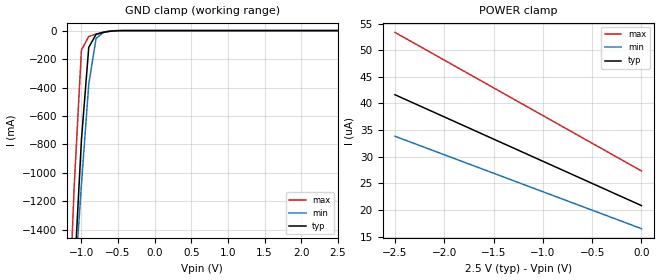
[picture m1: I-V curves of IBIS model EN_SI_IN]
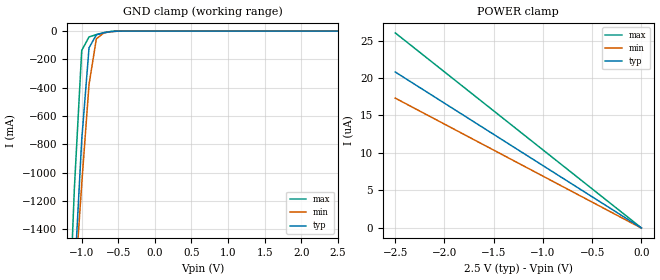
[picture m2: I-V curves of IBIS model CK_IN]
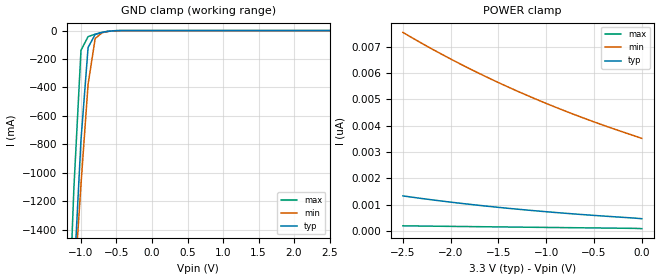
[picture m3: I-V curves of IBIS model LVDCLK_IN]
|   Texas Instruments Incorporated
|   IBIS Model for CDCLVD110A
|   32-PIN LQFP Package
[IBIS Ver]   3.2
[Comment char]   |_char
[File name]   cdclvd110a.ibs
[File Rev]   1.3   | pre-silicon, correlated to first silicon samples
[Date]   17Apr02
[Source]   File originated at Texas Instruments Incorporated.
   HPA HIGH SPEED COMMUNICATION AND CONTROLL, HSCC.
[Notes]   REVISION HISTORY:
   1.0: 03/26/02 initially release  version.
   1.1: 04/05/02 improved accuracy of rising/falling waveforms to solve
   warning messages during file check.
   Synchronized wave form data to match time with TPD
   (0ns = cross point at input)
   1.2: 04/17/02 Reviewed range completeness of I-V tables.
   1.3: 08/19/02 Corrected Warning on C_comp.
[Disclaimer]
(C) Copyright Texas Instruments Incorporated 2002
   All rights reserved
  Texas Instruments Incorporated hereby grants the user of this IBIS
model a non-exclusive, nontransferable license to use this IBIS model
under the following terms.  Before using this IBIS model, the user
should read this license.  If the user does not accept these terms,
the IBIS model should be returned to Texas Instruments within 30 days.
  The user is granted this license only to use the IBIS model and
is not granted rights to sell, load, rent, lease or license the IBIS
model in whole or in part, or in modified form to anyone other than
user.  User may modify the IBIS model to suit its specific applications
but rights to derivative works and such modifications shall belong to
Texas Instruments.
  This IBIS model is provided on an "AS IS" basis and Texas Instruments
makes absolutely no warranty with respect to the information contained
herein.  TEXAS INSTRUMENTS DISCLAIMS AND CUSTOMER WAIVES ALL WARRANTIES,
EXPRESS OR IMPLIED, INCLUDING WARRANTIES OF MERCHANTABILITY OR FITNESS
FOR A PARTICULAR PURPOSE. The entire risk as to quality and performance
is with the Customer. ACCORDINGLY, IN NO EVENT SHALL THE COMPANY BE LIABLE
FOR ANY DAMAGES, WHETHER IN CONTRACT OR TORT,INCLUDING ANY LOST PROFITS
OR OTHER INCIDENTAL, CONSEQUENTIAL, EXEMPLARY, OR PUNITIVE DAMAGES ARISING
OUT OF THE USE OR APPLICATION OF THE IBIS model provided in this package.
Further, Texas Instruments reserves the right to discontinue or make changes
without notice to any product herein to improve reliability, function, or
design. Texas Instruments does not convey any license under patent rights
or any other intellectual property rights, including those of third parties.
Contact Texas Instruments at ATTN: HPA-High Speed Communication & Control, HSCC
[Copyright]   Copyright 2002, Texas Instruments, All Rights Reserved
[Component]   CDCLVD110AVF
[Manufacturer]  Texas Instruments Incorporated
[Package]
|   typ   min   max
R_pkg   0.1026   0.0423   0.1248
L_pkg   3.424nH   2.117nH   4.030nH
C_pkg   0.276pF   0.217pF   0.610pF
[Pin] signal_name   model_name   R_pin   L_pin   C_pin
1   CK   CK_IN   0.1223   3.968nH   0.353pF
2   SI   EN_SI_IN   0.1106   3.670nH   0.268pF
3   CLK0_T   LVDCLK_IN   0.1043   3.429nH   0.235pF
4   CLK0_N   LVDCLK_IN   0.1018   3.304nH   0.218pF
5   VREF   NC   0.1022   3.313nH   0.218pF
6   CLK1_T   LVDCLK_IN   0.1054   3.453nH   0.228pF
7   CLK1_N   LVDCLK_IN   0.1129   3.696nH   0.247pF
8   EN   EN_SI_IN   0.1248   4.030nH   0.218pF
9   VSS   GND   0.0621   2.573nH   0.514pF
10   Q9_N   LVDCLK_OUT   0.1132   3.725nH   0.261pF
11   Q9_T   LVDCLK_OUT   0.1072   3.492nH   0.235pF
12   Q8_N   LVDCLK_OUT   0.1048   3.371nH   0.219pF
13   Q8_T   LVDCLK_OUT   0.1053   3.380nH   0.221pF
14   Q7_N   LVDCLK_OUT   0.1083   3.516nH   0.230pF
15   Q7_T   LVDCLK_OUT   0.1148   3.750nH   0.253pF
16   VDD   POWER   0.0424   2.117nH   0.476pF
17   Q6_N   LVDCLK_OUT   0.1235   3.997nH   0.288pF
18   Q6_T   LVDCLK_OUT   0.1116   3.673nH   0.265pF
19   Q5_N   LVDCLK_OUT   0.1048   3.439nH   0.234pF
20   Q5_T   LVDCLK_OUT   0.1020   3.309nH   0.219pF
21   Q4_N   LVDCLK_OUT   0.1020   3.308nH   0.217pF
22   Q4_T   LVDCLK_OUT   0.1047   3.440nH   0.227pF
23   Q3_N   LVDCLK_OUT   0.1115   3.690nH   0.250pF
24   Q3_T   LVDCLK_OUT   0.1232   3.995nH   0.284pF
25   VSS   GND   0.0423   2.117nH   0.610pF
26   Q2_N   LVDCLK_OUT   0.1151   3.751nH   0.258pF
27   Q2_T   LVDCLK_OUT   0.1082   3.517nH   0.236pF
28   Q1_N   LVDCLK_OUT   0.1052   3.381nH   0.219pF
29   Q1_T   LVDCLK_OUT   0.1048   3.371nH   0.219pF
30   Q0_N   LVDCLK_OUT   0.1071   3.493nH   0.227pF
31   Q0_T   LVDCLK_OUT   0.1131   3.728nH   0.256pF
32   VDD   POWER   0.0621   2.572nH   0.422pF
| 'T' (true) pin is non-inverted Diff_pin and the
| 'N' (negate) pin is the inverted Diff_pin
[Diff_pin]   inv_pin   vdiff   tdelay_typ   tdelay_min   tdelay_max
   3   4   0.2V   NA
   6   7   0.2V   NA
   11   10   NA   NA
   13   12   NA   NA
   15   14   NA   NA
   18   17   NA   NA
   20   19   NA   NA
   22   21   NA   NA
   24   23   NA   NA
   27   26   NA   NA
   29   28   NA   NA
   31   30   NA   NA
| Models and submodels in the file (4): EN_SI_IN (Input), CK_IN (Input), LVDCLK_IN (Input), LVDCLK_OUT (Output)
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|   EN- AND SI-INPUT Model
[Model]   EN_SI_IN
Model_type   Input
|Signals   EN,SI
Vinh = 2.0
Vinl = 0.8
|   typ   min   max
C_comp   1.1pF   NA   NA
|   typ   min   max
[Temperature Range]   50   105   -40
[Voltage range]   2.5V   2.375V   2.625V
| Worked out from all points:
|   GND clamp passes 1 mA (typ) near -0.52 V on its own axis
|TEMP refers to junction temp.
[GND_clamp]
|  Voltage   I(typ)   I(min)   I(max)
-2.5V     -15.75A    -12.62A    -19.3A
-1.2V     -2.748A    -2.615A    -2.404A
-1.1V     -1.749A    -1.846A    -1.108A
-1V       -768.5mA   -1.08A     -136.8mA
-900mV    -117.8mA   -376.9mA   -41.31mA
-800mV    -26.27mA   -54.64mA   -24.52mA
-700mV    -12.17mA   -13.75mA   -11.2mA
-600mV    -3.967mA   -4.581mA   -2.699mA
-400mV    -49.11uA   -105uA     -9.81uA
2.5V      20.81uA    17.35uA    26.02uA
[Power_clamp]
| Note that the[POWER_clamp]voltage table is referenced to Vcc
| and is calculated using Vtable=Vcc - Vmeasured.
|  Voltage   I(typ)   I(min)   I(max)
-2.5V     41.63uA    33.83uA    53.34uA
-1.1V     29.97uA    24.11uA    38.77uA
-800mV    27.48uA    22.03uA    35.65uA
0V        20.81uA    16.48uA    27.32uA
|   CK-INPUT Model
[Model]   CK_IN
Model_type   Input
|Signals   CK
Vinh = 2.0
Vinl = 0.8
|   typ   min   max
C_comp   2.9pF   NA   NA
|   typ   min   max
[Temperature Range]   50   105   -40
[Voltage range]   2.5V   2.375V   2.625V
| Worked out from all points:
|   GND clamp passes 1 mA (typ) near -0.52 V on its own axis
|TEMP refers to junction temp.
[GND_clamp]
|  Voltage   I(typ)   I(min)   I(max)
-2.5V     -15.75A    -12.62A    -19.3A
-1.2V     -2.748A    -2.615A    -2.404A
-1.1V     -1.749A    -1.846A    -1.108A
-1V       -768.5mA   -1.08A     -136.8mA
-900mV    -117.9mA   -376.9mA   -41.33mA
-800mV    -26.28mA   -54.65mA   -24.54mA
-700mV    -12.18mA   -13.76mA   -11.22mA
-600mV    -3.984mA   -4.594mA   -2.722mA
-400mV    -69.79uA   -121.3uA   -37.1uA
2.5V      -14.49nA   834.9nA    -1.301uA
[Power_clamp]
| Note that the[POWER_clamp]voltage table is referenced to Vcc
| and is calculated using Vtable=Vcc - Vmeasured.
|  Voltage   I(typ)   I(min)   I(max)
-2.5V     20.8uA     17.32uA    26.02uA
-1.9V     15.81uA    13.15uA    19.77uA
-1.8V     14.97uA    12.46uA    18.73uA
0V        -14.49nA   -32.51nA   -24.8pA
|   LVD110 CLOCK Input MODEL
[Model]   LVDCLK_IN
Model_type   Input
|Signals   CLK0_T,CLK0_N,CLK1_T,CLK1_N
Vinh = 1.35
Vinl = 1.15
|   typ   min   max
C_comp   2.9pF   NA   NA
|   typ   min   max
[Temperature Range]   50   105   -40
[Voltage range]   3.3V   3.0V   3.6V
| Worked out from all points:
|   GND clamp passes 1 mA (typ) near -0.51 V on its own axis
[GND_clamp]
|   Voltage   I(typ)   I(min)   I(max)
-2.5V     -15.75A    -12.62A    -19.31A
-1.2V     -2.749A    -2.616A    -2.406A
-1.1V     -1.75A     -1.847A    -1.11A
-1V       -769.8mA   -1.081A    -138.5mA
-900mV    -119mA     -377.9mA   -42.58mA
-800mV    -27.04mA   -55.44mA   -25.33mA
-700mV    -12.59mA   -14.19mA   -11.61mA
-600mV    -4.13mA    -4.764mA   -2.815mA
-400mV    -48.29uA   -107.8uA   -5.963uA
2.5V      466.4pA    3.676nA    76.09pA
[Power_clamp]
| Note that the[POWER_clamp]voltage table is referenced to Vcc
| and is calculated using Vtable=Vcc - Vmeasured.
|   Voltage   I(typ)   I(min)   I(max)
-2.5V     1.334nA    7.552nA    196.4pA
-2.2V     1.187nA    6.93nA     183.7pA
-1.9V     1.054nA    6.351nA    171.3pA
-1.6V     935.5pA    5.814nA    159.2pA
-1.3V     828.5pA    5.314nA    147.2pA
-1V       732.3pA    4.85nA     135.4pA
-700mV    645.6pA    4.419nA    123.8pA
-400mV    567.4pA    4.018nA    112.2pA
0V        466.4pA    3.52nA     88.41pA
